(* Logix 5000 AddOnInstructionDefinition export D_SHL; software revision 30.00 *)

ADD_ON_INSTRUCTION D_SHL   (* revision 1.0 20170524, vendor Kenneth A. Fischer *)
// DINT bit shift left of the 32-bit argument Inp_A by Inp_B bits with paddding by zeros on the right
// Revision note:
// Rev1.0: 20170524 - Initial Release
VAR_IN_OUT
   Inp_A : DINT; {required}   // 64-bit Integer to be right circular rotated
END_VAR
VAR_INPUT
   Inp_B : INT; {required}   // Number of bits to shift
END_VAR
VAR_IN_OUT
   Out : DINT; {required}   // Result
END_VAR
VAR
   Wrk_InpA : DINT[2];
   Source_Bit : BOOL;
   ONS : BOOL;
   BSL_Cntrl : CONTROL := (LEN := 32);
END_VAR

ROUTINE Logic   (* ladder *)
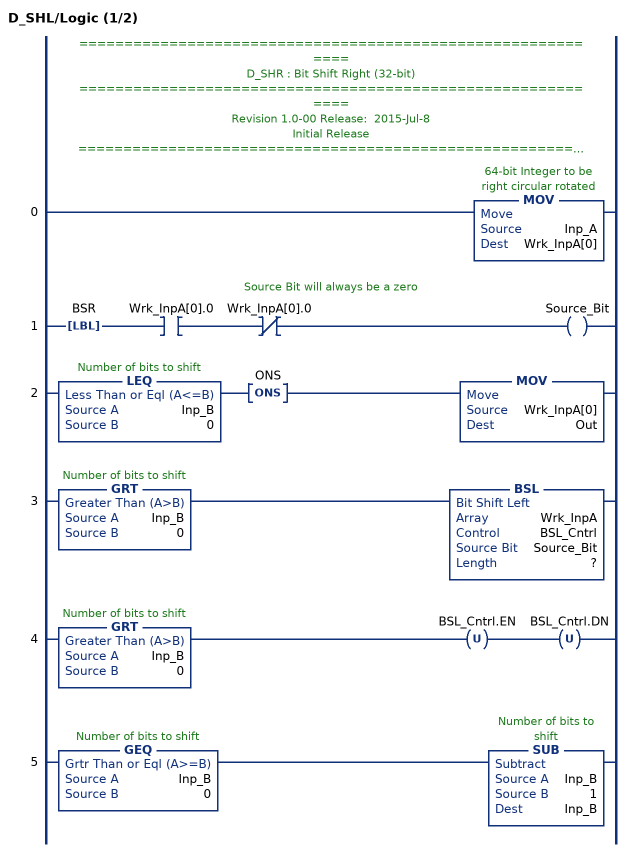
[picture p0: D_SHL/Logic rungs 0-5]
   // ============================================================
   // D_SHR : Bit Shift Right (32-bit)
   // ============================================================
   // Revision 1.0-00 Release:  2015-Jul-8
   // Initial Release
   // ============================================================
   // Performs a left bit shift of the 32-bit argument Inp_A by the
   // number of bits defined in the 16-bit argument Inp_B, with padding by zeros.
   0: MOV(Inp_A,Wrk_InpA[0]);
   // Source Bit will always be a zero
   1: LBL(BSR)XIC(Wrk_InpA[0].0)XIO(Wrk_InpA[0].0)OTE(Source_Bit);
   2: LEQ(Inp_B,0)ONS(ONS)MOV(Wrk_InpA[0],Out);
   3: GRT(Inp_B,0)BSL(Wrk_InpA,BSL_Cntrl,Source_Bit,?);
   4: GRT(Inp_B,0)OTU(BSL_Cntrl.EN)OTU(BSL_Cntrl.DN);
   5: GEQ(Inp_B,0)SUB(Inp_B,1,Inp_B);
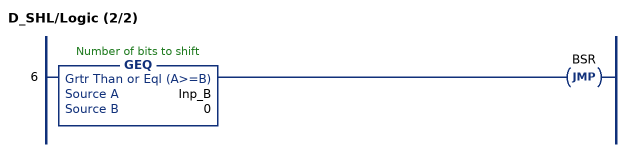
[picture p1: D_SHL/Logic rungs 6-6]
   6: GEQ(Inp_B,0)JMP(BSR);
END_ROUTINE
END_ADD_ON_INSTRUCTION
